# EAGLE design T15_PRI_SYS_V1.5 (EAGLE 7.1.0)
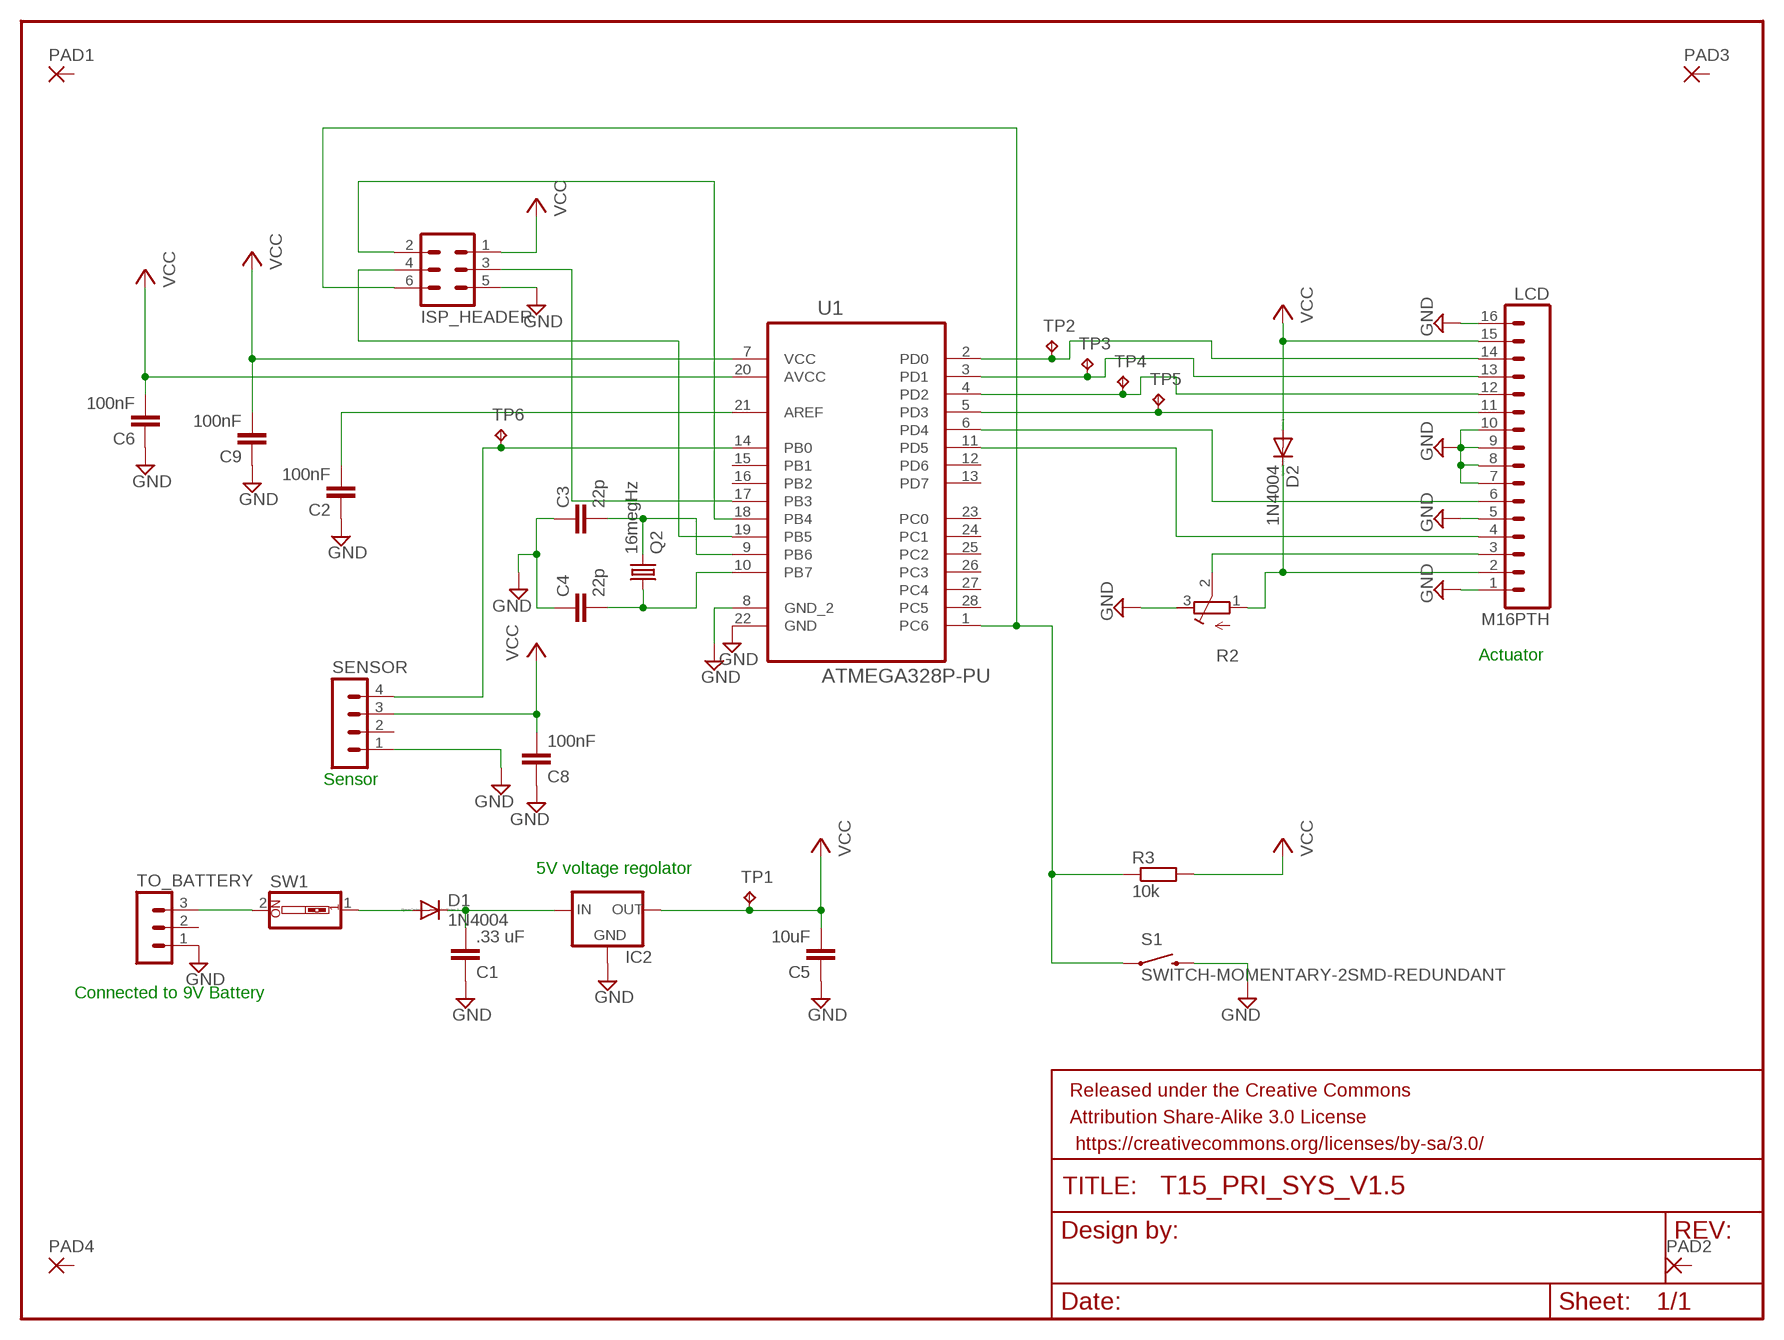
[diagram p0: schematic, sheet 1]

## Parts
C1  .33 uF  C-EU025-024X044  [C025-024X044]
C2  100nF  C-EU025-024X044  [C025-024X044]
C3  22p  C-EU025-024X044  [C025-024X044]
C4  22p  C-EU025-024X044  [C025-024X044]
C5  10uF  C-EU025-024X044  [C025-024X044]
C6  100nF  C-EU025-024X044  [C025-024X044]
C8  100nF  C-EU025-024X044  [C025-024X044]
C9  100nF  C-EU025-024X044  [C025-024X044]
D1  1N4004  [DO41-10]
D2  1N4004  [DO41-10]
FRAME1  FRAME-LETTER  [CREATIVE_COMMONS]
IC2  78XXL  [78XXL]
ISP_HEADER  MA03-2  [MA03-2]
LCD  M16PTH  [1X16]
PAD1  1,6/0,8  [1,6/0,8]
PAD2  1,6/0,8  [1,6/0,8]
PAD3  1,6/0,8  [1,6/0,8]
PAD4  1,6/0,8  [1,6/0,8]
Q2  16megHz  CRYSTALHC49S  [HC49/S]
R2  R-TRIMMTS63Z  [RTRIMTS63Z]
R3  10k  R-EU_0204/5  [0204/5]
S1  SWITCH-MOMENTARY-2SMD-REDUNDANT  [TACTILE-SWITCH-SMD]
SENSOR  MA04-1  [MA04-1]
SW1  SW_DIP-1  [EDG-01]
TO_BATTERY  MA03-1  [MA03-1]
TP1  TPB1,27  [B1,27]
TP2  TPB1,27  [B1,27]
TP3  TPB1,27  [B1,27]
TP4  TPB1,27  [B1,27]
TP5  TPB1,27  [B1,27]
TP6  TPB1,27  [B1,27]
U1  ATMEGA328P-PU  [DIP254P762X457-28]

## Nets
GND: C1.1 C2.1 C3.1 C4.1 C5.1 C6.1 C8.1 C9.1 IC2.GND ISP_HEADER.5 LCD.1 LCD.5 LCD.7 LCD.8 LCD.9 LCD.10 LCD.16 R2.3(E) S1.3 S1.4 SENSOR.1 TO_BATTERY.1 U1.8(GND_2) U1.22(GND)
MISO: ISP_HEADER.2 U1.18(PB4)
MOSI: ISP_HEADER.3 U1.17(PB3)
N$2: D2.C LCD.2 R2.1(A)
N$3: LCD.3 R2.2(S)
N$5: C1.2 D1.C IC2.IN
N$8: C3.2 Q2.2 U1.9(PB6)
N$9: LCD.11 TP5.TP U1.5(PD3)
N$10: C4.2 Q2.1 U1.10(PB7)
N$11: LCD.12 TP4.TP U1.4(PD2)
N$12: LCD.13 TP3.TP U1.3(PD1)
N$13: LCD.14 TP2.TP U1.2(PD0)
N$14: SW1.2 TO_BATTERY.3
N$17: LCD.6 U1.6(PD4)
N$18: LCD.4 U1.11(PD5)
N$20: D1.A SW1.1
PBO: SENSOR.4 TP6.TP U1.14(PB0)
RESET: ISP_HEADER.6 R3.1 S1.1 S1.2 U1.1(PC6)
SCK: ISP_HEADER.4 U1.19(PB5)
VCC: C5.2 C6.2 C8.2 C9.2 D2.A IC2.OUT ISP_HEADER.1 LCD.15 R3.2 SENSOR.3 TP1.TP U1.7(VCC) U1.20(AVCC)
VCC1: C2.2 U1.21(AREF)
Unconnected: PAD1.1(P) PAD2.1(P) PAD3.1(P) PAD4.1(P) SENSOR.2 TO_BATTERY.2 U1.12(PD6) U1.13(PD7) U1.15(PB1) U1.16(PB2) U1.23(PC0) U1.24(PC1) U1.25(PC2) U1.26(PC3) U1.27(PC4) U1.28(PC5)

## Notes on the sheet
- Actuator
- Sensor
- 5V voltage regolator
- Connected to 9V Battery

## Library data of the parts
C1-C6 C8 C9 = rcl:C-EU: CAPACITOR, European symbol
D1 D2 = diode:1N4004: DIODE
FRAME1 = SparkFun-Retired:FRAME-LETTER: Schematic Frame
IC2 = v-reg:78XXL: VOLTAGE REGULATOR
ISP_HEADER = con-lstb:MA03-2: PIN HEADER; OC_FARNELL: unknown; OC_NEWARK: unknown
LCD = SparkFun-Connectors:M16: 1x16 .1" header
PAD1-PAD4 = wirepad:1,6/0,8: THROUGH-HOLE PAD
Q2 = crystal:CRYSTAL: CRYSTAL; OC_FARNELL: 1667008; OC_NEWARK: unknown
R2 = rcl:R-TRIMM: Trimm resistor
R3 = rcl:R-EU_: RESISTOR, European symbol
S1 = SparkFun-Electromechanical:SWITCH-MOMENTARY-2: Various NO switches- pushbuttons, reed, etc
SENSOR = con-lstb:MA04-1: PIN HEADER; OC_FARNELL: unknown; OC_NEWARK: unknown
SW1 = special:SW_DIP-1: DIP SWITCH
TO_BATTERY = con-lstb:MA03-1: PIN HEADER; OC_FARNELL: unknown; OC_NEWARK: unknown
TP1-TP6 = testpad:TP: Test pad
U1 = Atmel_By_element14_Batch_1-00:ATMEGA328P-PU: 8-bit Microcontroller with In-System Programmable Flash; MPN: ATMEGA328P-PU; OC_FARNELL: 1715487; OC_NEWARK: 15R0268; PACKAGE: PDIP-28; SUPPLIER: Atmel

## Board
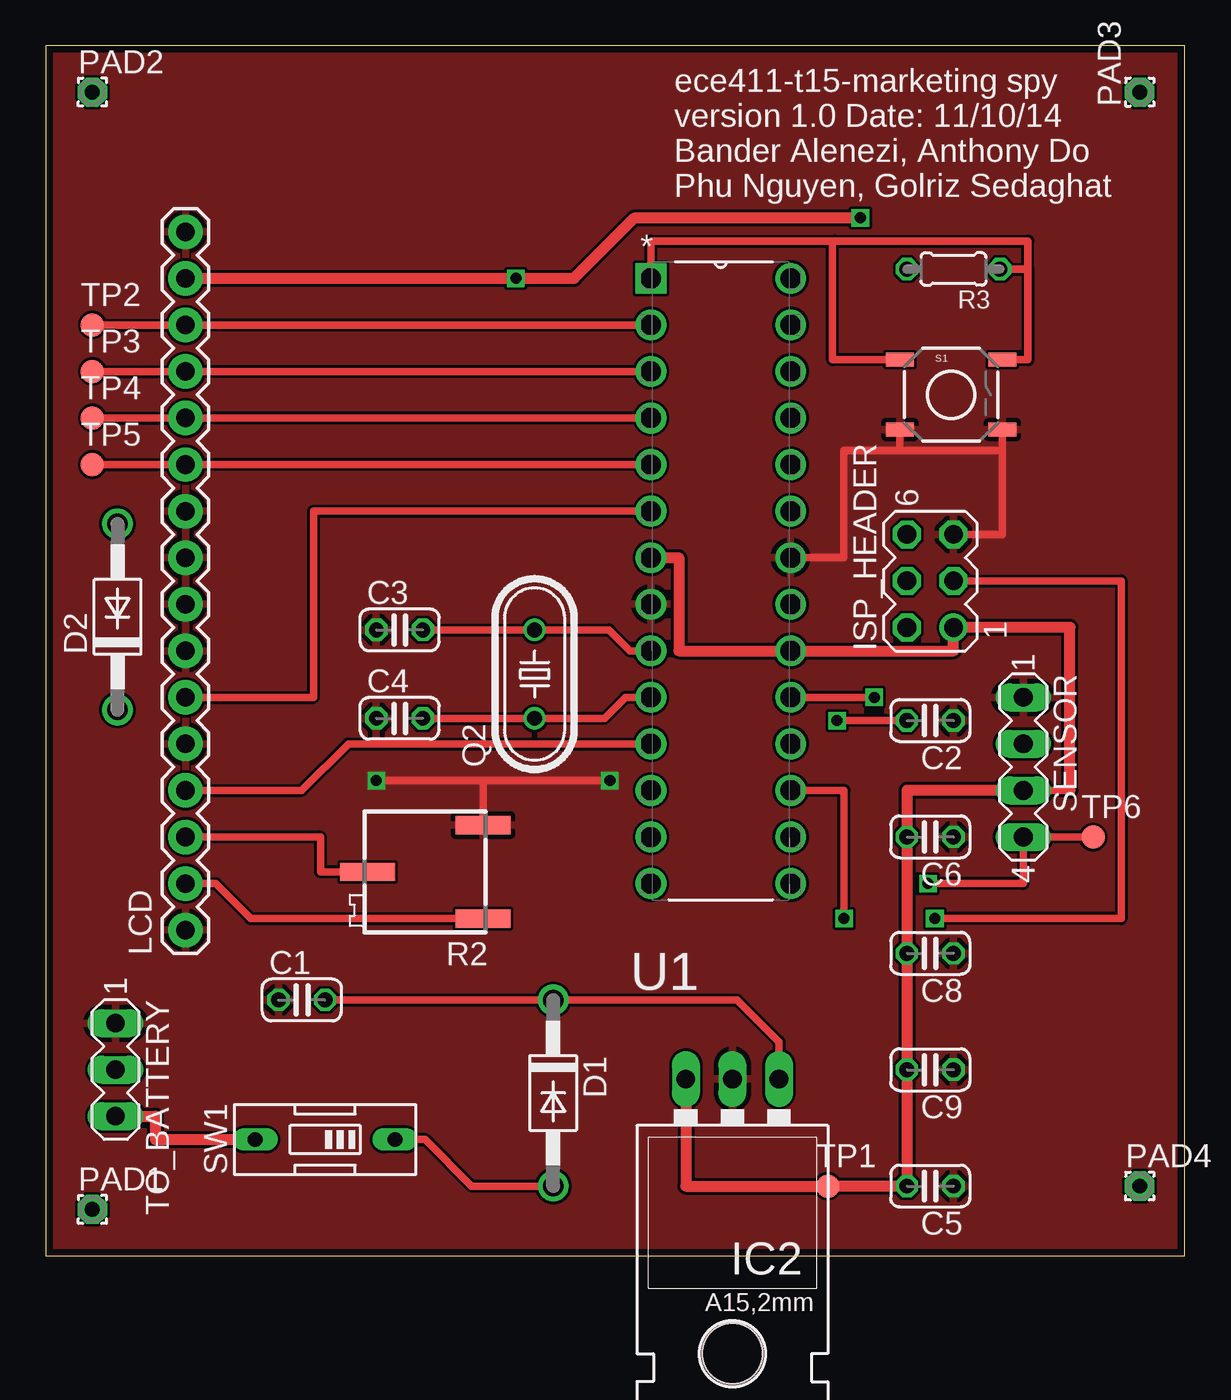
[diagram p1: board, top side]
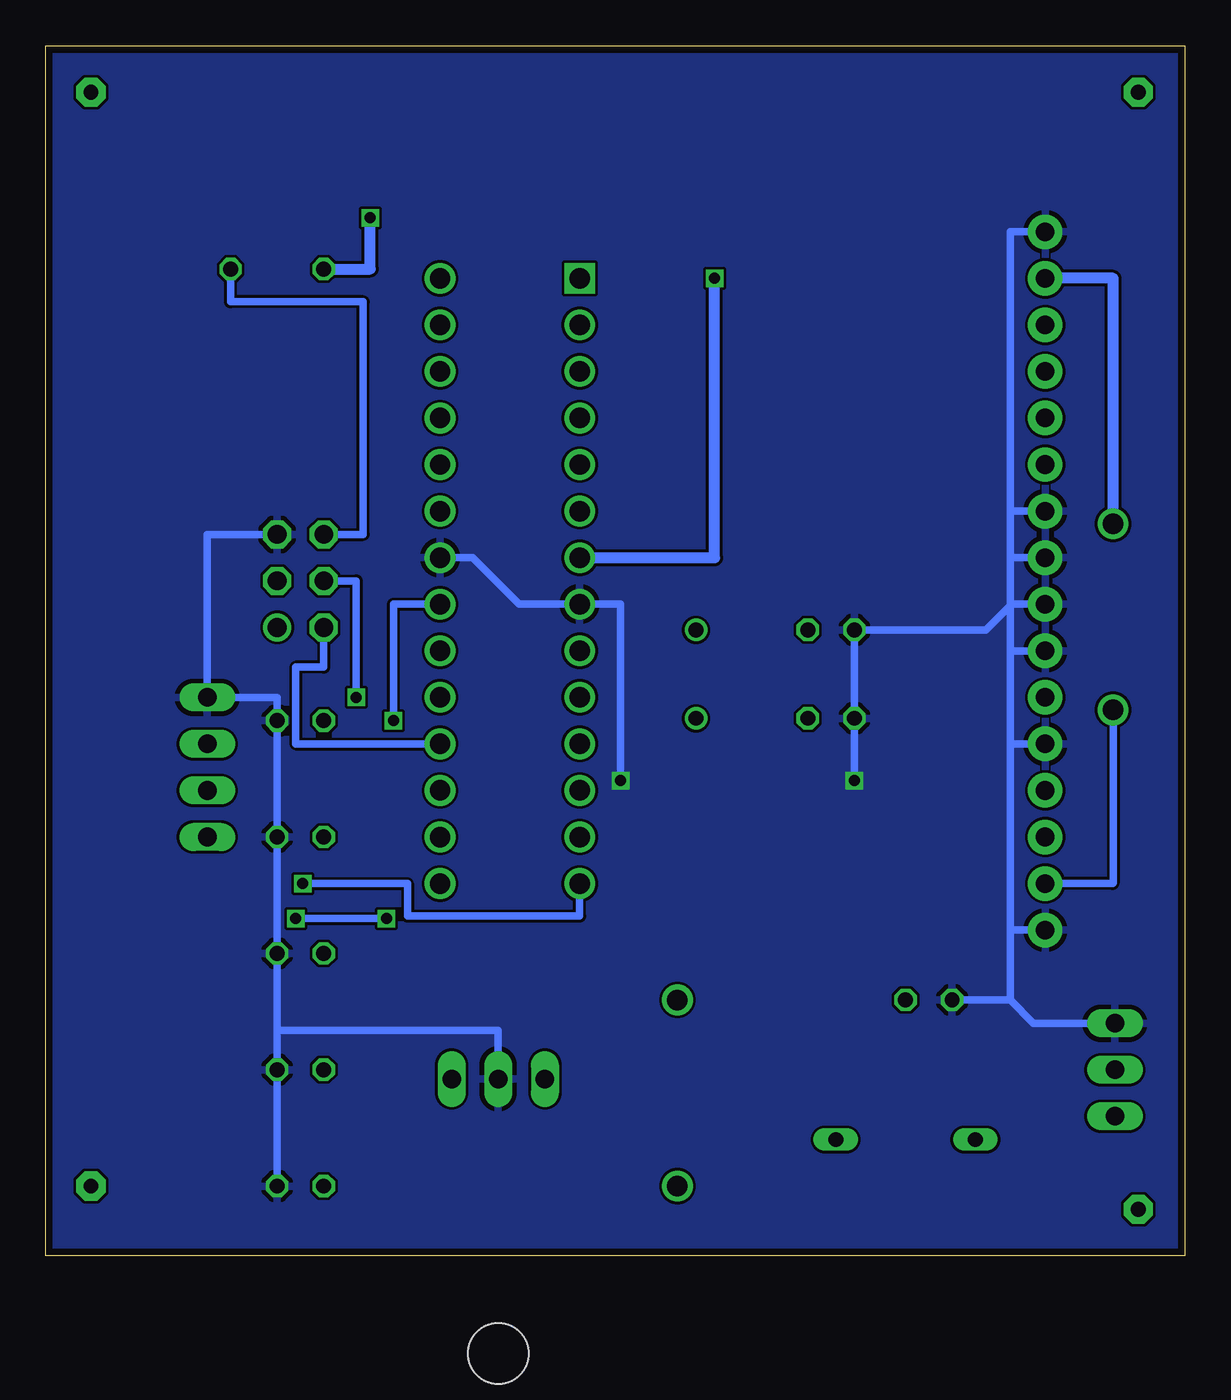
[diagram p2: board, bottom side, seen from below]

Size 62.15 x 66.03 mm. Coordinates in mm from the lower left corner, seen from the top.
Outline: 0,0 62.15,0 62.15,66.03 0,66.03 0,0
Copper layers (1*16): Top 0.0356mm / dielectric 1.5011mm / Bottom 0.0356mm
Design rules "DRC": minimum track width 6mil, minimum drill 13mil, track to track 6mil, track to pad 6mil, pad to pad 6mil, via to via 6mil, smd to smd 6mil, copper to edge 15mil, drill to drill 6mil, minimum pad ring 7mil, minimum via ring 7mil, stop-mask expansion 3mil, vias tented up to drill 0mil, thermal gap 10mil

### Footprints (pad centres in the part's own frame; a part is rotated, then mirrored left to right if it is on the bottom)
C025-024X044 = drill 0.813 octagon: 1 -1.27,0; 2 1.27,0
DO41-10 = drill 1.118: A 5.08,0; C -5.08,0
78XXL = drill 1.016 long: GND 0,-3.81; IN -2.54,-3.81; OUT 2.54,-3.81 | hole 3.302: 0,11.176
MA03-2 = drill 1.016: 1 -2.54,-1.27 | drill 1.016 octagon: 2 -2.54,1.27; 3 0,-1.27; 4 0,1.27; 5 2.54,-1.27; 6 2.54,1.27
1X16 = drill 1.016 pad 1.88: 1 0,0; 2 2.54,0; 3 5.08,0; 4 7.62,0; 5 10.16,0; 6 12.7,0; 7 15.24,0; 8 17.78,0; 9 20.32,0; 10 22.86,0; 11 25.4,0; 12 27.94,0; 13 30.48,0; 14 33.02,0; 15 35.56,0; 16 38.1,0
1,6/0,8 = drill 0.813 pad 1.6 octagon: 1 0,0
HC49/S = drill 0.813: 1 -2.413,0; 2 2.413,0
RTRIMTS63Z = smd 1 x 3: 1 -2.55,-3.15; 2 0,3.15; 3 2.55,-3.15
0204/5 = drill 0.813 octagon: 1 -2.54,0; 2 2.54,0
TACTILE-SWITCH-SMD = smd 1.524 x 0.762: 1 -2.794,1.905; 2 2.794,1.905; 3 -2.794,-1.905; 4 2.794,-1.905
MA04-1 = drill 1.016 long: 1 -3.81,0; 2 -1.27,0; 3 1.27,0; 4 3.81,0
EDG-01 = drill 0.813 long: 1 0,-3.81; 2 0,3.81
MA03-1 = drill 1.016 long: 1 -2.54,0; 2 0,0; 3 2.54,0
B1,27 = smd 1.27 x 1.27: TP 0,0
DIP254P762X457-28 = drill 1.118 square: 1 -7.62,33.02 | drill 1.118: 2 -7.62,30.48; 3 -7.62,27.94; 4 -7.62,25.4; 5 -7.62,22.86; 6 -7.62,20.32; 7 -7.62,17.78; 8 -7.62,15.24; 9 -7.62,12.7; 10 -7.62,10.16; 11 -7.62,7.62; 12 -7.62,5.08; 13 -7.62,2.54; 14 -7.62,0; 15 0,0; 16 0,2.54; 17 0,5.08; 18 0,7.62; 19 0,10.16; 20 0,12.7; 21 0,15.24; 22 0,17.78; 23 0,20.32; 24 0,22.86; 25 0,25.4; 26 0,27.94; 27 0,30.48; 28 0,33.02

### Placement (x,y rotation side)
C1  13.97,13.97 0 top
C2  48.26,29.21 180 top
C3  19.3,34.16 0 top
C4  19.3,29.34 0 top
C5  48.26,3.81 180 top
C6  48.26,22.86 180 top
C8  48.26,16.51 180 top
C9  48.26,10.16 180 top
D1  27.69,8.89 270 top
D2  3.91,34.87 90 top
FRAME1  not placed on the board
IC2  37.47,5.84 180 top
ISP_HEADER  48.26,36.83 90 top
LCD  7.62,17.78 90 top
PAD1  2.54,2.54 0 top
PAD2  2.54,63.5 0 top
PAD3  59.69,63.5 90 top
PAD4  59.69,3.81 0 top
Q2  26.67,31.75 90 top
R2  20.7,20.95 90 top
R3  49.53,53.85 180 top
S1  49.4,46.99 0 top
SENSOR  53.34,26.67 270 top
SW1  15.24,6.35 90 top
TO_BATTERY  3.81,10.16 270 top
TP1  42.67,3.81 0 top
TP2  2.54,50.8 0 top
TP3  2.54,48.26 0 top
TP4  2.54,45.72 0 top
TP5  2.54,43.18 0 top
TP6  57.15,22.86 0 top
U1  40.64,20.32 0 top

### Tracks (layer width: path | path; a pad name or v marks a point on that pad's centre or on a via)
GND  (via drill 0.6)
  Top 0.406: S1.4 52.2,43.94 | 52.2,43.94 46.61,43.94 | 46.61,43.94 S1.3 | ISP_HEADER.5 52.2,39.37 52.2,43.94 | U1.22 43.56,38.1 43.56,43.94 46.61,43.94 | v18.03,25.93 23.85,25.93 | 23.85,25.93 R2.3 | R2.3 | v30.79,25.93 23.85,25.93
  Bottom 0.406: LCD.16 9.53,55.88 9.53,40.64 | LCD.10 9.53,40.64 | 9.53,40.64 9.53,38.1 | LCD.9 9.53,38.1 | 9.53,38.1 9.53,35.56 | LCD.8 9.53,35.56 | 9.53,35.56 9.53,35.48 | 9.53,35.48 9.53,33.02 | LCD.7 9.53,33.02 | 9.53,33.02 9.53,27.94 | LCD.5 9.53,27.94 | 9.53,27.94 9.53,17.78 | LCD.1 9.53,17.78 | 9.53,17.78 9.53,13.97 | 9.53,13.97 C1.1 | TO_BATTERY.1 8.26,12.7 9.53,13.97 | ISP_HEADER.5 53.34,39.37 SENSOR.1 49.53,30.48 C2.1 C6.1 C8.1 49.53,12.32 | 49.53,12.32 C9.1 C5.1 | IC2.GND 37.47,12.32 49.53,12.32 | U1.22 38.86,38.1 36.32,35.56 U1.8 30.79,35.56 v30.79,25.93 | v18.03,25.93 C4.1 C3.1 10.85,34.16 9.53,35.48
  pour Bottom: -1.27,67.31 63.5,67.31 63.5,-1.27 -1.27,-1.27
  pour Top: -1.27,67.31 63.5,67.31 63.5,-1.27 -1.27,-1.27
  pour Bottom: -1.27,67.31 63.5,67.31 63.5,-1.27 -1.27,-1.27 -1.27,66.04
MISO
  Bottom 0.406: U1.18 48.51,27.94 48.51,32.13 46.99,32.13 ISP_HEADER.2
MOSI  (via drill 0.6)
  Top 0.406: ISP_HEADER.3 58.67,36.83 58.67,18.41 v48.51,18.41 | v43.56,18.41 43.56,25.4 U1.17
  Bottom 0.406: v48.51,18.41 v43.56,18.41
N$2
  Top 0.406: LCD.2 9.27,20.32 11.18,18.41 23.84,18.41 R2.1
  Bottom 0.406: D2.C 3.91,20.34 3.94,20.32 LCD.2
N$3
  Top 0.406: R2.2 14.99,20.95 14.99,22.86 LCD.3
N$5
  Top 0.406: C1.2 D1.C 37.72,13.97 40.01,11.68 IC2.IN
N$8
  Top 0.406: U1.9 31.88,33.02 30.73,34.16 Q2.2 C3.2
N$9
  Top 0.406: U1.5 LCD.11 TP5.TP
N$10
  Top 0.406: U1.10 31.62,30.48 30.48,29.34 Q2.1 C4.2
N$11
  Top 0.406: U1.4 LCD.12 TP4.TP
N$12
  Top 0.406: U1.3 LCD.13 TP3.TP
N$13
  Top 0.406: U1.2 LCD.14 TP2.TP
N$14
  Top 0.61: TO_BATTERY.3 5.97,7.62 5.97,6.35 SW1.2
N$17
  Top 0.406: LCD.6 14.61,30.48 14.61,40.64 U1.6
N$18
  Top 0.406: LCD.4 13.97,25.4 16.51,27.94 U1.11
N$20
  Top 0.406: D1.A 23.24,3.81 20.7,6.35 SW1.1
PBO  (via drill 0.6)
  Top 0.406: TP6.TP SENSOR.4 53.34,20.32 v48.13,20.32
  Bottom 0.406: v48.13,20.32 42.42,20.32 42.42,18.54 33.02,18.54 U1.14
RESET
  Top 0.406: R3.1 53.59,53.85 | 53.59,53.85 53.59,55.37 43.05,55.37 | 53.59,53.85 53.59,48.9 S1.2 | U1.1 33.02,55.37 43.05,55.37 | S1.1 42.93,48.9 42.93,55.24 43.05,55.37
  Bottom 0.406: ISP_HEADER.6 44.83,39.37 44.83,52.07 52.07,52.07 R3.1
SCK  (via drill 0.6)
  Top 0.406: v45.21,30.48 U1.19
  Bottom 0.406: ISP_HEADER.4 45.21,36.83 v45.21,30.48
VCC  (via drill 0.6)
  Top 0.406: SENSOR.3 55.88,25.4
  Top 0.61: LCD.15 v25.65,53.34 28.83,53.34 32.13,56.64 v44.45,56.64 | U1.7 34.54,38.1 34.54,33.02 U1.20 49.53,33.02 ISP_HEADER.1 55.88,34.29 55.88,25.4 | SENSOR.3 46.99,25.4 C6.2 C8.2 C9.2 C5.2 TP1.TP 34.92,3.81 IC2.OUT
  Bottom 0.61: R3.2 44.45,53.85 v44.45,56.64 | D2.A 3.91,53.34 LCD.15 | U1.7 25.65,38.1 v25.65,53.34
VCC1  (via drill 0.6)
  Top 0.406: C2.2 v43.18,29.21
  Bottom 0.406: v43.18,29.21 43.18,35.56 U1.21

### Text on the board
tNames: ece411-t15-marketing spy / version 1.0 Date: 11/10/14 / Bander Alenezi, Anthony Do / Phu Nguyen, Golriz Sedaghat

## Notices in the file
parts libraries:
SparkFun-Retired: Licensing:Creative Commons ShareAlike 4.0 International - https://creativecommons.org/licenses/by-sa/4.0
SparkFun-Retired: Released under the Creative Commons Attribution Share-Alike 3.0 License
SparkFun-Retired: https://creativecommons.org/licenses/by-sa/3.0
